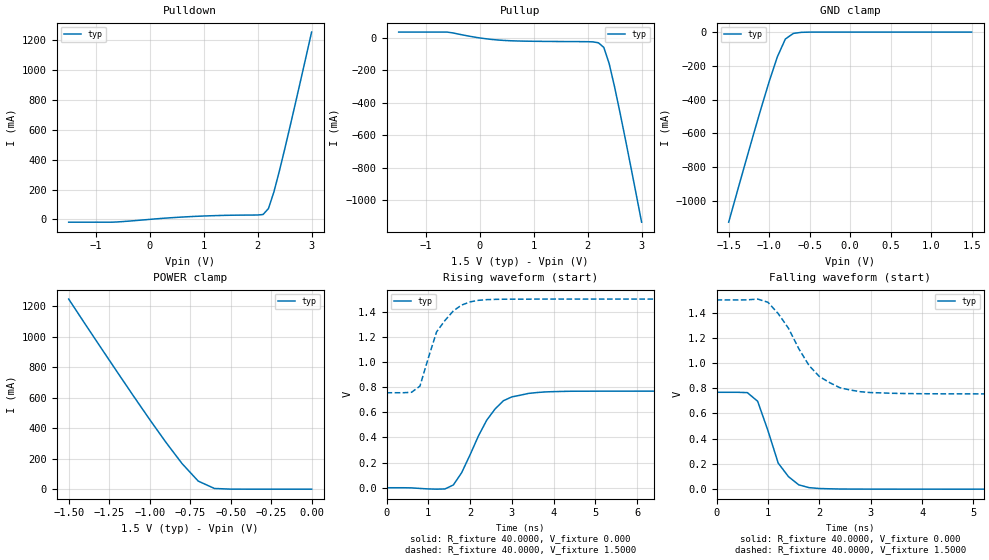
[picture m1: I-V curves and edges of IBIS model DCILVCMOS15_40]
| / 7\'7
| \ \   Xilinx Inc.
| / /
| \_\/.\   IBIS Model for Virtex-II
[IBIS ver]   2.1
[File name]   dci1540.ibs
[File Rev]   1.1
[Date]   Aug. 1, 2001
[Source]   Hspice simulations (08-01: TT, SS, FF)
[Notes]   Xilinx IBIS model for LVDCI 1.5V 40 ohms driver
[Disclaimer] The data in this model is derived from SPICE simulations using
   modeling information extracted from the target process. While
   a great deal of care has been taken to provide information
   that is accurate, this model is considered preliminary as it
   has not been verified by actual silicon measurement. Treat the
   data in this model as preliminary until actual silicon
   verification is performed.
[Copyright]   Copyright 2001, Xilinx Inc., All rights reserved
|   Component Virtex_II
[Component]   Virtex_II
[Manufacturer]   Xilinx Inc.
[Package]
| variable   typ   min   max
R_pkg   0.1000   NA   NA
L_pkg   0.8000nH   NA   NA
C_pkg   0.5000pF   NA   NA
[Pin]  signal_name   model_name   R_pin   L_pin   C_pin
io   DCILVCMOS15_40   DCILVCMOS15_40
| ins  insig   inp
| ens  ensig   inp
PGND   GND   GND
VCCO   VCCO   POWER
| Models and submodels in the file (1): DCILVCMOS15_40 (I/O)
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|   Model DCILVCMOS15_40
[Model]   DCILVCMOS15_40
Model_type   I/O
Polarity   Non-Inverting
Enable   Active-Low
Vinh = 1.05V
Vinl = 0.3V
Vmeas =   0.7300V
Cref =  35.0000pF
Rref =   1.0000M
Vref =  0.000V
C_comp   7.0000pF   NA   NA
[Temperature Range]   25.0000   NA   NA
[Voltage Range]   1.5000V   NA   NA
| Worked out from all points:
|   slope of the pulldown table from 0 to 0.225 V, typ, clamps not added: 34.1 ohm
|   slope of the pullup table from 0 to 0.225 V, typ, clamps not added: 24.1 ohm
|   GND clamp passes 1 mA (typ) near -0.57 V on its own axis
|   POWER clamp passes 1 mA (typ) near -0.52 V on its own axis
|   rising waveform, R_fixture 40.0000, V_fixture 0.000: 20-80 % time 726ps typ, NA min, NA max; typ from 0 V to 0.768 V
|   rising waveform, R_fixture 40.0000, V_fixture 1.5000: 20-80 % time 569ps typ, NA min, NA max; typ from 0.755 V to 1.5 V
|   falling waveform, R_fixture 40.0000, V_fixture 0.000: 20-80 % time 427ps typ, NA min, NA max; typ from 0.768 V to 0 V
|   falling waveform, R_fixture 40.0000, V_fixture 1.5000: 20-80 % time 705ps typ, NA min, NA max; typ from 1.5 V to 0.755 V
[Pulldown]
| voltage   I(typ)   I(min)   I(max)
-1.5V     -18.84mA   NA         NA
-700mV    -18.84mA   NA         NA
700mV     17.59mA    NA         NA
2.1V      32.6mA     NA         NA
2.2V      72.23mA    NA         NA
2.3V      181.9mA    NA         NA
2.4V      320.2mA    NA         NA
2.5V      468.6mA    NA         NA
2.7V      778.5mA    NA         NA
3V        1.256A     NA         NA
[Pullup]
| voltage   I(typ)   I(min)   I(max)
-1.5V     35.85mA    NA         NA
-600mV    35.85mA    NA         NA
0V        -8.2nA     NA         NA
500mV     -16.43mA   NA         NA
2V        -23.25mA   NA         NA
2.2V      -30.04mA   NA         NA
2.3V      -58.39mA   NA         NA
2.4V      -159.3mA   NA         NA
2.5V      -302.6mA   NA         NA
2.6V      -460.5mA   NA         NA
2.8V      -793mA     NA         NA
3V        -1.135A    NA         NA
[GND_clamp]
| voltage   I(typ)   I(min)   I(max)
-1.5V     -1.127A    NA         NA
-1.2V     -617mA     NA         NA
-1V       -293.4mA   NA         NA
-900mV    -148mA     NA         NA
-800mV    -41mA      NA         NA
-700mV    -7.588mA   NA         NA
-600mV    -1.413mA   NA         NA
1.5V      218.4nA    NA         NA
[POWER_clamp]
| voltage   I(typ)   I(min)   I(max)
-1.5V     1.246A     NA         NA
-1.1V     610.9mA    NA         NA
-900mV    307.7mA    NA         NA
-800mV    167.8mA    NA         NA
-700mV    52.78mA    NA         NA
-600mV    4.607mA    NA         NA
0V        218.4nA    NA         NA
[Ramp]
| variable   typ   min   max
dV/dt_r   0.4608/0.7116n   NA   NA
dV/dt_f   0.4468/0.6627n   NA   NA
R_load = 40.0000
[Rising Waveform]
R_fixture = 40.0000
V_fixture = 0.000
| time   V(typ)   V(min)   V(max)
0s        6.363uV    NA         NA
1.4ns     -9.707mV   NA         NA
1.6ns     22.08mV    NA         NA
1.8ns     120.1mV    NA         NA
2.4ns     537.2mV    NA         NA
2.8ns     691.9mV    NA         NA
3ns       722.2mV    NA         NA
3.6ns     756.8mV    NA         NA
4.4ns     767.1mV    NA         NA
10ns      768mV      NA         NA
[Rising Waveform]
R_fixture = 40.0000
V_fixture = 1.5000
V_fixture_min = 1.4000
V_fixture_max = 1.6000
| time   V(typ)   V(min)   V(max)
0s        755.3mV    NA         NA
600ps     759mV      NA         NA
800ps     807.9mV    NA         NA
1.2ns     1.24V      NA         NA
1.6ns     1.406V     NA         NA
1.8ns     1.452V     NA         NA
2ns       1.478V     NA         NA
2.4ns     1.496V     NA         NA
2.8ns     1.499V     NA         NA
10ns      1.5V       NA         NA
[Falling Waveform]
R_fixture = 40.0000
V_fixture = 0.000
| time   V(typ)   V(min)   V(max)
0s        768mV      NA         NA
600ps     765.2mV    NA         NA
800ps     697mV      NA         NA
1ns       465mV      NA         NA
1.2ns     206.6mV    NA         NA
1.4ns     99.26mV    NA         NA
1.6ns     34.33mV    NA         NA
1.8ns     12.14mV    NA         NA
2.6ns     722uV      NA         NA
10ns      58.4uV     NA         NA
[Falling Waveform]
R_fixture = 40.0000
V_fixture = 1.5000
V_fixture_min = 1.4000
V_fixture_max = 1.6000
| time   V(typ)   V(min)   V(max)
0s        1.5V       NA         NA
800ps     1.507V     NA         NA
1ns       1.482V     NA         NA
1.4ns     1.276V     NA         NA
1.8ns     980.4mV    NA         NA
2ns       893.5mV    NA         NA
2.2ns     844.7mV    NA         NA
2.6ns     786.4mV    NA         NA
4ns       756.6mV    NA         NA
10ns      755.3mV    NA         NA
